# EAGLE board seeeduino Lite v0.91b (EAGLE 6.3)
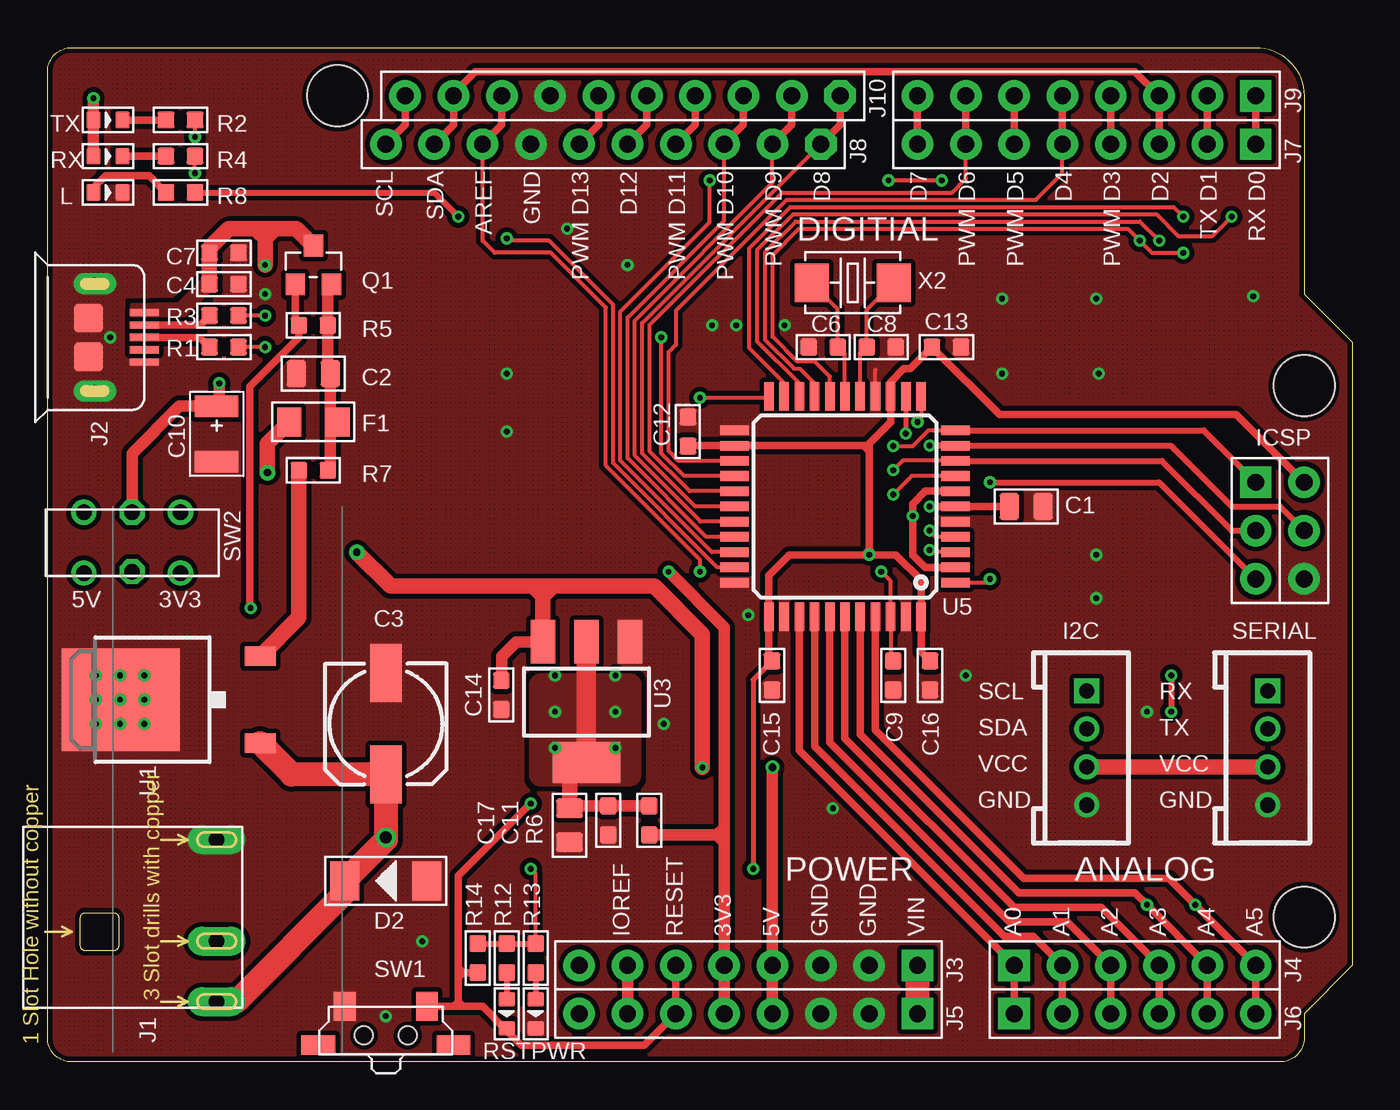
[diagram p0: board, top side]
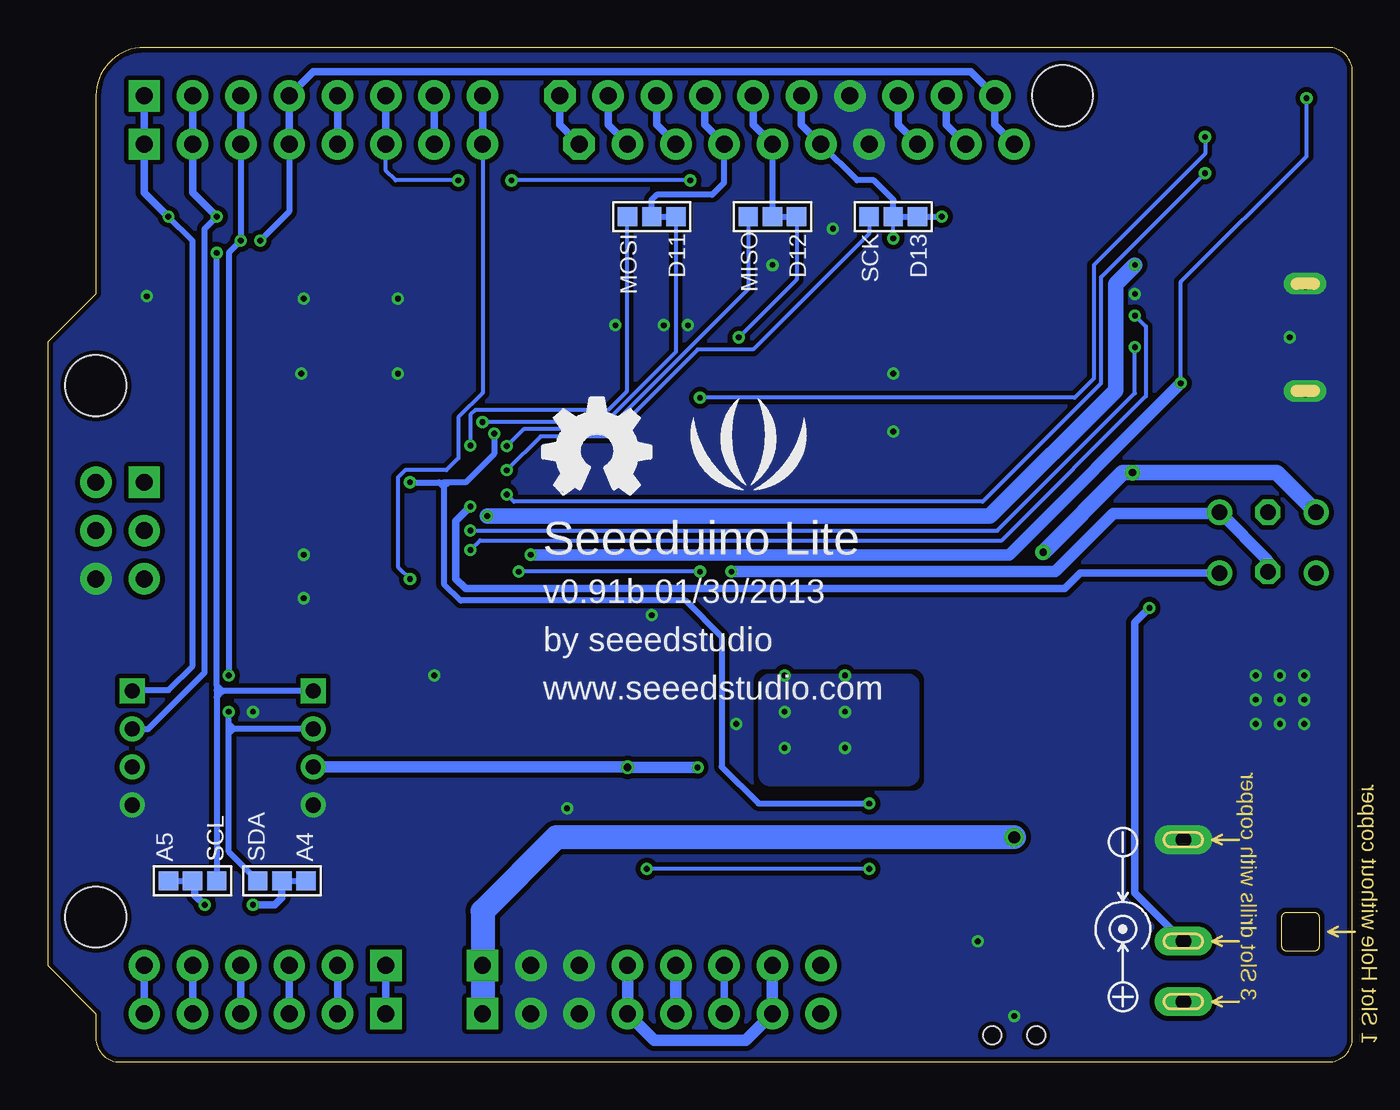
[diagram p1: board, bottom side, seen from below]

Size 68.58 x 53.34 mm. Coordinates in mm from the lower left corner, seen from the top.
Outline: 66.04,2.54 66.04,1.27 arc-90 64.77,0 1.27,0 arc-90 0,1.27 0,52.07 arc-90 1.27,53.34 63.5,53.34 arc-90 66.04,50.8 66.04,40.39 68.58,37.85 68.58,5.08 66.04,2.54
Copper layers (1*16): Top 0.035mm / dielectric 1.5mm / Bottom 0.035mm
Design rules "default *": minimum track width 6mil, minimum drill 12mil, track to track 6mil, track to pad 6mil, pad to pad 6mil, via to via 6mil, smd to smd 0mil, copper to edge 10mil, drill to drill 10mil, minimum pad ring 10mil, minimum via ring 6mil, stop-mask expansion 2mil, vias tented up to drill 100mil, thermal gap 10mil
Net classes: 0 default: width 0.152 mm, drill 0.305 mm, clearance 0.152 mm; 3 none3: width 0.203 mm, drill 0.305 mm, clearance 0.203 mm
Holes 3.2 mm at 15.24,50.8 66.04,35.56 66.04,7.62

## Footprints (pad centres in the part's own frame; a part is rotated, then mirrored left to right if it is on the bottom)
C0805 = smd 1.016 x 1.397: 1 -0.889,0; 2 0.889,0
ELECTRO-SMD-C-6MM = smd 3.048 x 1.651: + 2.667,0; - -2.667,0
C0603 = smd 0.889 x 0.889: 1 -0.762,0; 2 0.762,0
AVX-B = smd 1.143 x 2.286: + -1.46,0; - 1.46,0
D2010 = smd 1.524 x 2.032: + -2.159,0; - 2.159,0
F1206 = smd 1.27 x 1.524: 1 -1.27,0; 2 1.27,0
4P-LEADED-2.0 = drill 0.8 pad 1.27 square: 1 -3,0 | drill 0.8 pad 1.27: 2 -1,0; 3 1,0; 4 3,0
2X3P-2.54 = drill 0.889 pad 1.651 square: 1 -1.27,2.54 | drill 0.889 pad 1.651: 2 -1.27,0; 3 -1.27,-2.54; 4 1.27,-2.54; 5 1.27,0; 6 1.27,2.54
DC-404 = drill 0.813 pad 1.524 long: + 3.175,10.16; - -5.334,10.16; CDN 0,10.16
MICRO-USB-5P = smd 0.38 x 1.52: 1 -1.3,0; 2 -0.65,0; 3 0,0; 4 0.65,0; 5 1.3,0 | smd 1.524 x 1.524: E1 -1.016,-2.921; E2 1.016,-2.921 | drill 0.635 pad 1.143 long: P1 -2.819,-2.591; P2 2.819,-2.591
8P-2.54-65/35MIL = drill 0.889 pad 1.651 square: 1 0,8.89 | drill 0.889 pad 1.651: 2 0,6.35; 3 0,3.81; 4 0,1.27; 5 0,-1.27; 6 0,-3.81; 7 0,-6.35; 8 0,-8.89
6P-2.54-65/35MIL = drill 0.889 pad 1.651 square: 1 0,6.35 | drill 0.889 pad 1.651: 2 0,3.81; 3 0,1.27; 4 0,-1.27; 5 0,-3.81; 6 0,-6.35
10P-2.54 = drill 0.889 pad 1.651 octagon: 1 0,11.43 | drill 0.889 pad 1.651: 2 0,8.89; 3 0,6.35; 4 0,3.81; 5 0,1.27; 6 0,-1.27; 7 0,-3.81; 8 0,-6.35; 9 0,-8.89; 10 0,-11.43
LED-0603 = smd 0.762 x 0.889: + -0.762,0; - 0.762,0
3P-SMD-4.1X1.5 = smd 1.016 x 1.016: 00 -1.27,0; 11 1.27,0; MM 0,0
SOT23 = smd 1.016 x 1.143: 1 -0.95,-1.016; 2 0.95,-1.016; 3 0,1.016
R0603 = smd 0.889 x 0.889: 1 -0.762,0; 2 0.762,0
4P-SMD-7X3.5X3.5H = smd 1.143 x 1.524: 1 -2.159,1.524; 2 2.159,1.524 | smd 1.778 x 1.016: S1 -3.556,-0.508; S2 3.556,-0.508 | hole 0.95: -1.15,0; 1.15,0
6P-2CH-2.5-9.1X3.5X3.2H = drill 0.813 pad 1.27: CH1A -2.54,-1.6; CH1B 2.54,-1.6; CH2A -2.54,1.6; CH2B 2.54,1.6 | drill 0.813 pad 1.27 octagon: COM1 0,-1.6; COM2 0,1.524
TO252 = smd 1.016 x 1.651: 1 -2.286,-4.826; 2 2.286,-4.826 | smd 5.4 x 6.2: 3 0,2.5
SOT-223 = smd 1.27 x 2.286: 1 -2.286,-3.175; 2 0,-3.175; 3 2.286,-3.175 | smd 3.556 x 2.159: TER 0,3.175
TQFP44 = smd 1.5 x 0.5: 1 -5.8,4; 2 -5.8,3.2; 3 -5.8,2.4; 4 -5.8,1.6; 5 -5.8,0.8; 6 -5.8,0; 7 -5.8,-0.8; 8 -5.8,-1.6; 9 -5.8,-2.4; 10 -5.8,-3.2; 11 -5.8,-4; 23 5.8,-4; 24 5.8,-3.2; 25 5.8,-2.4; 26 5.8,-1.6; 27 5.8,-0.8; 28 5.8,0; 29 5.8,0.8; 30 5.8,1.6; 31 5.8,2.4; 32 5.8,3.2; 33 5.8,4 | smd 0.5 x 1.5: 12 -4,-5.8; 13 -3.2,-5.8; 14 -2.4,-5.8; 15 -1.6,-5.8; 16 -0.8,-5.8; 17 0,-5.8; 18 0.8,-5.8; 19 1.6,-5.8; 20 2.4,-5.8; 21 3.2,-5.8; 22 4,-5.8; 34 4,5.8; 35 3.2,5.8; 36 2.4,5.8; 37 1.6,5.8; 38 0.8,5.8; 39 0,5.8; 40 -0.8,5.8; 41 -1.6,5.8; 42 -2.4,5.8; 43 -3.2,5.8; 44 -4,5.8
2P-SMD-5X3.2 = smd 1.778 x 2.032: 1 -2.159,0; 2 2.159,0

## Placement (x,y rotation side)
C1  1uF  [C0805]  51.44,29.21 180 top
C2  10uF  [C0805]  13.97,36.2 180 top
C3  25v_47uF  [ELECTRO-SMD-C-6MM]  17.78,17.78 270 top
C4  100nF  [C0603]  9.27,40.89 0 top
C6  8.2pF  [C0603]  40.77,37.59 0 top
C7  10nF  [C0603]  9.27,42.55 0 top
C8  8.2pF  [C0603]  43.81,37.59 180 top
C9  100nF  [C0603]  44.45,20.32 90 top
C10  47uF 10V  [AVX-B]  8.89,33.02 270 top
C11  100nF  [C0603]  29.46,12.7 90 top
C12  100nF  [C0603]  33.66,33.15 270 top
C13  100nF  [C0603]  47.24,37.59 180 top
C14  100nF  [C0603]  23.85,19.3 90 top
C15  100nF  [C0603]  38.07,20.32 90 top
C16  100nF  [C0603]  46.38,20.32 90 top
C17  10uF  [C0805]  27.43,12.45 90 top
D2  M7  [D2010]  17.78,9.53 180 top
F1  PPTC-500mA  [F1206]  13.97,33.66 180 top
I2C  4P-LEADED-2.0  [4P-LEADED-2.0]  54.61,16.51 270 top
ICSP  2.54-2x3p male  [2X3P-2.54]  64.77,27.94 0 top
J1  DC-044-AH  [DC-404]  -1.27,6.35 270 top
J2  USB-MICRO-5P  [MICRO-USB-5P]  5.08,38.1 270 top
J3  DNP  [8P-2.54-65/35MIL]  36.83,5.08 270 top
J4  DNP  [6P-2.54-65/35MIL]  57.15,5.08 90 top
J5  2.54-6p female  [8P-2.54-65/35MIL]  36.83,2.54 270 top
J6  2.54-6p female  [6P-2.54-65/35MIL]  57.15,2.54 90 top
J7  DNP  [8P-2.54-65/35MIL]  54.61,48.26 270 top
J8  DNP  [10P-2.54]  29.21,48.26 270 top
J9  2.54-8p female  [8P-2.54-65/35MIL]  54.61,50.8 270 top
J10  2.54-8p female  [10P-2.54]  30.23,50.8 270 top
L  GREEN  [LED-0603]  3.17,45.72 0 top
MISO  DNP  [3P-SMD-4.1X1.5]  30.48,44.45 0 bottom
MOSI  DNP  [3P-SMD-4.1X1.5]  36.83,44.45 0 bottom
PWR  GREEN  [LED-0603]  25.65,2.54 270 top
Q1  Si2305Ds  [SOT23]  13.97,41.91 0 top
R1  22R  [R0603]  9.27,37.59 0 top
R2  1k  [R0603]  6.99,49.53 180 top
R3  22R  [R0603]  9.27,39.24 0 top
R4  1k  [R0603]  6.99,47.62 180 top
R5  100k  [R0603]  13.97,38.73 0 top
R6  0R  [R0603]  31.62,12.7 270 top
R7  0R  [R0603]  13.97,31.11 0 top
R8  1k  [R0603]  6.99,45.72 0 top
R12  1k  [R0603]  24.13,5.46 270 top
R13  1k  [R0603]  25.65,5.46 270 top
R14  10k  [R0603]  22.61,5.46 270 top
RST  RED  [LED-0603]  24.13,2.54 270 top
RX  GREEN  [LED-0603]  3.17,47.62 0 top
SCK  DNP  [3P-SMD-4.1X1.5]  24.13,44.45 0 bottom
SCL  DNP  [3P-SMD-4.1X1.5]  60.96,9.53 0 bottom
SDA  DNP  [3P-SMD-4.1X1.5]  56.26,9.53 180 bottom
SERIAL  4P-LEADED-2.0  [4P-LEADED-2.0]  64.14,16.51 270 top
SW1  BUTTON-4P-REINFORCE'TS-118E'  [4P-SMD-7X3.5X3.5H]  17.78,1.4 0 top
SW2  SWITCH-2CH-6P-2.54  [6P-2CH-2.5-9.1X3.5X3.2H]  4.45,27.3 180 top
TX  GREEN  [LED-0603]  3.17,49.53 0 top
U1  78M05-TO252  [TO252]  6.35,19.05 90 top
U3  LD1117S  [SOT-223]  28.32,18.92 180 top
U5  ATMEGA32U4-AU  [TQFP44]  41.91,29.21 180 top
U$1  [OSHW_FILLX200_NOTEXT]  42.55,29.84 0 bottom
U$2  [LOGO_SILK]  31.75,31.75 0 bottom
X2  16MHz  [2P-SMD-5X3.2]  42.32,40.97 180 top

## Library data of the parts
C1-C4 C6-C17 D2 F1 L PWR Q1 R1-R8 R12-R14 RST RX SW1 SW2 TX X2 = Discrete
I2C ICSP J2-J10 SERIAL = Connector
J1 = For_Test_Albert
MISO MOSI SCK SCL SDA = Discrete; PARTNO: DNP
U1 U3 U5 = IC
U$1 U$2 = Logo

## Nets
3V3: J3.5 J5.5 R6.2 SW2.CH1A SW2.COM2
5V [none3]: C14.2 F1.2 I2C.3 J3.4 J3.7 J5.4 J5.7 SERIAL.3 SW2.CH1B U3.3
AREF: C9.2 J8.8 J10.8 U5.42
D14/PB3/MISO: ICSP.1 MISO.00 U5.11
D15/PB1/SCK: ICSP.2 SCK.00 U5.9
D16/PB2/MOSI: ICSP.5 MOSI.00 U5.10
D17/PB0/RXLED: R4.1 U5.8
D+: R1.2 U5.4
D-: R3.2 U5.3
GATE: J1.CDN Q1.1 R5.1
GND [none1]: C1.1 C2.2 C3.- C4.2 C6.1 C7.2 C8.1 C9.1 C10.- C11.1 C12.1 C13.1 C14.1 C15.1 C16.1 C17.1 D2.+ I2C.4 ICSP.4 J1.- J2.5 J2.E1 J2.E2 J2.P1 J2.P2 J3.2 J3.3 J5.2 J5.3 J8.7 J10.7 L.- PWR.- SERIAL.4 SW1.1 U1.3 U3.1 U5.5 U5.15 U5.23 U5.33 U5.35 U5.43
N$1: C6.2 U5.17 X2.2
N$2: C8.2 U5.16 X2.1
N$3: C11.2 C17.2 R6.1 U3.2 U3.TER
N$4: L.+ R8.1
N$5: R2.2 TX.-
N$6: J2.2 R3.1
N$7: R4.2 RX.-
N$8: J2.3 R1.1
N$9: C2.1 F1.1 Q1.2 R5.2 R7.2
N$10: PWR.+ R13.2
N$11: R7.1 U1.2
N$17: R12.2 RST.+
PB4/A8/D8: J8.1 J10.1 U5.28
PB5/A9/D9: J8.2 J10.2 U5.29
PB6/A10/D10: J8.3 J10.3 U5.30
PB7/D11: J8.4 J10.4 MOSI.11 MOSI.MM U5.12
PC7/D13: J8.6 J10.6 R8.2 SCK.11 SCK.MM U5.32
PD0/SCL/D3: I2C.1 J7.4 J8.10 J9.4 J10.10 SCL.11 U5.18
PD1/SDA/D2: I2C.2 J7.3 J8.9 J9.3 J10.9 SDA.11 U5.19
PD2/RXI/D0: J7.1 J9.1 SERIAL.1 U5.20
PD3/TXO/D1: J7.2 J9.2 SERIAL.2 U5.21
PD4/A6/D4: J7.5 J9.5 U5.25
PD5/TXLED: R2.1 U5.22
PD6/A11/D12: J8.5 J10.5 MISO.11 MISO.MM U5.26
PD6/D5: J7.6 J9.6 U5.31
PD7/A7/D6: J7.7 J9.7 U5.27
PE6/D7: J7.8 J9.8 U5.1
PF0/A5: J4.6 J6.6 SCL.00 SCL.MM U5.41
PF1/A4: J4.5 J6.5 SDA.00 SDA.MM U5.40
PF4/A3: J4.4 J6.4 U5.39
PF5/A2: J4.3 J6.3 U5.38
PF6/A1: J4.2 J6.2 U5.37
PF7/A0: J4.1 J6.1 U5.36
PWR_IN: C3.+ D2.- J1.+ J3.1 J5.1 U1.1
RESET: ICSP.3 J3.6 J5.6 R14.2 RST.- SW1.2 U5.13
U5V: C4.1 C7.1 J2.1 Q1.3 U5.2 U5.7
UCAP: C1.2 SW2.CH2A U5.6
VCC: C10.+ C12.2 C13.2 C15.2 C16.2 ICSP.6 R12.1 R13.1 R14.1 RX.+ SW2.COM1 TX.+ U5.14 U5.24 U5.34 U5.44

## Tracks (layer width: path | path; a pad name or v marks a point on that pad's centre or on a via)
3V3  (via drill 0.3 pad 0.64)
  Top 0.61: J5.5 J3.5 35.56,11.56 | v32.64,25.78 35.56,22.86 35.56,12.32 | 35.56,11.81 35.56,12.32 | R6.2 35.18,11.94 | 35.18,11.94 35.43,11.94 35.56,11.81 | 35.18,11.94 35.56,12.32 | 35.18,11.94 35.56,11.56 | 35.56,11.56 35.56,11.81
  Bottom 0.61: SW2.COM2 4.45,26.36 SW2.CH1A arc90 7.06,28.83 12.57,28.83 15.62,25.78 v32.64,25.78 | J5.5 J3.5
5V  (via drill 0.3 pad 0.64, 0.38 pad 0.81, 0.41)
  Top 0.61: J5.4 J3.4 v38.1,15.49 | U3.3 24.64,22.1 23.88,21.34 23.88,20.09 C14.2 | J3.7 J5.7
  Top 0.813: SERIAL.3 I2C.3 | F1.2 11.56,32.51 v11.56,30.99 | v16.26,26.8 18.03,25.02 25.53,25.02 | 25.53,25.02 26.16,25.02 | 26.16,25.02 26.04,24.89 26.04,24.51 | 26.04,24.51 26.04,24.38 | 26.04,24.38 U3.3 | 26.04,24.38 arc45 25.95,24.6 25.53,25.02 | 26.16,25.02 31.88,25.02 34.42,22.48 v34.42,15.49 | 26.04,24.51 26.42,24.89
  Bottom 0.61: I2C.3 38.12,15.51 v38.1,15.49 v34.42,15.49 | J5.7 31.88,1.14 36.7,1.14 J5.4 J3.4 | J3.7 30.48,2.67
  Bottom 0.813: SW2.CH1B 3.99,30.99 v11.56,30.99 12.06,30.99 v16.26,26.8
AREF  (via drill 0.3 pad 0.64)
  Top 0.203: 44.31,21.22 U5.42 44.31,25.29 v43.81,25.78 | J8.8 22.86,43.18 23.5,42.55 26.46,42.55 29.34,39.67 29.34,31.37 34.29,26.42 v34.29,25.78
  Top 0.305: 44.31,21.22 C9.2
  Top 0.406: J10.8 23.88,49.28 J8.8
  Bottom 0.203: v34.29,25.78 v43.81,25.78
  Bottom 0.406: J10.8 23.88,49.28 J8.8
D14/PB3/MISO  (via drill 0.3 pad 0.64)
  Top 0.203: 47.65,33.27 U5.11 46.29,33.21 45.47,32.38 v44.45,32.38
  Top 0.305: U5.11 60.77,33.21 ICSP.1
  Bottom 0.203: MISO.00 31.75,40.64 39.12,33.27 43.56,33.27 v44.45,32.38
D15/PB1/SCK  (via drill 0.3 pad 0.64)
  Top 0.203: 47.57,31.75 47.7,31.62 | 47.7,31.62 U5.9 | 47.7,31.62 44.96,31.62 v44.45,31.11
  Top 0.305: U5.9 58.56,31.61 62.23,27.94 ICSP.2
  Bottom 0.203: 25.4,44.07 SCK.00 25.4,43.56 31.5,37.47 34.42,37.47 38.99,32.89 42.67,32.89 v44.45,31.11
D16/PB2/MOSI  (via drill 0.3 pad 0.64)
  Top 0.305: U5.10 v46.35,32.41 59.03,32.41 62.23,29.21 64.77,29.21 ICSP.5
  Bottom 0.203: MOSI.00 arc-45 38.14,44.43 38.14,35.26 39.12,34.29 46.1,34.29 46.35,34.04 v46.35,32.41
D17/PB0/RXLED  (via drill 0.3 pad 0.64)
  Top 0.203: U5.8 45.41,30.81 v44.45,29.84 | v7.75,46.74 R4.1
  Bottom 0.203: v44.45,29.84 44.07,29.46 19.43,29.46 13.21,35.69 13.21,41.27 v7.75,46.74
D+  (via drill 0.3 pad 0.64)
  Top 0.203: U5.4 46.69,27.61 v46.35,27.94 | v11.43,37.59 R1.2
  Bottom 0.203: v46.35,27.94 18.66,27.94 11.43,35.17 v11.43,37.59
D-  (via drill 0.3 pad 0.64)
  Top 0.203: U5.3 46.47,26.81 v46.35,26.92 | v11.43,39.24 R3.2
  Bottom 0.203: v46.35,26.92 45.85,27.43 18.43,27.43 10.86,35 10.86,38.67 v11.43,39.24
GATE  (via drill 0.3 pad 0.64)
  Top 0.406: Q1.1 13.02,38.92 R5.1 | R5.1 13.08,38.73 | R5.1 13.21,38.1 10.63,35.52 10.63,23.91 v10.67,23.88
  Bottom 0.406: J1.CDN 11.43,8.89 11.43,23.11 v10.67,23.88
GND  (via drill 0.3 pad 0.64)
  Top 0.203: U5.15 43.51,36.4
  other vias: 50.16,36.2 55.24,36.2 50.16,40.13 41.27,13.34 36.83,23.5 11.43,40.39 30.48,41.91 57.78,18.41 55.12,40.13 63.37,40.26 24.13,36.2 24.13,33.15 3.3,38.1 19.68,6.35 17.78,2.41 48.26,20.32 55.12,26.67 55.12,24.38 32.38,17.78 34.92,38.73 2.54,20.32 5.08,20.32 5.08,17.78 2.54,17.78 27.3,43.81 38.73,38.73 36.2,38.73 5.08,19.05 2.54,19.05 3.81,20.32 3.81,19.05 3.81,17.78
  pour Bottom (isolate 0.254, rank 2, no thermals): 0,0 66.04,0 66.04,2.54 68.58,5.08 68.58,37.85 66.04,40.39 66.04,51.82 64.52,53.34 0,53.34
  pour Top (isolate 0.254, rank 2, no thermals, hatched): 0,0 66.04,0 66.04,2.54 68.58,5.08 68.58,37.85 66.04,40.39 66.04,51.82 64.52,53.34 0,53.34
N$1
  Top 0.203: X2.2 41.53,39.6 C6.2 41.91,37.21 U5.17
N$2
  Top 0.203: U5.16 42.71,37.25 C8.2 43.05,39.55 X2.1
N$3  (via drill 0.3 pad 0.64)
  Top 0.305: 27.43,15.62 28.19,15.62 U3.TER
  Top 0.61: C17.2 27.56,13.46 C11.2 R6.1
  Top 0.813: C17.2 27.43,15.62
  Top 1.016: U3.TER U3.2
  other vias: 26.67,20.32 26.67,16.51 29.84,16.51 29.84,18.41 26.67,18.41 29.84,20.32
  pour Bottom (isolate 0.254, no thermals): 22.86,19.81 22.86,15.11 arc90 23.37,14.61 30.61,14.61 arc90 31.11,15.11 31.11,19.81 arc90 30.61,20.32 23.37,20.32 arc90
  pour Top (isolate 0.254, no thermals): 25.4,19.81 25.4,15.11 arc90 25.91,14.61 30.61,14.61 arc90 31.11,15.11 31.11,19.81 arc90 30.61,20.32 25.91,20.32 arc90
N$4
  Top 0.406: L.+ 2.41,45.97 3.05,46.61 5.33,46.61 R8.1
N$5
  Top 0.406: TX.- R2.2
N$6
  Top 0.406: J2.2 8.02,38.75 R3.1
N$7
  Top 0.406: R4.2 RX.-
N$8
  Top 0.406: J2.3 8,38.1 R1.1
N$9
  Top 0.406: 14.92,38.92 R5.2 | 14.86,34.04 F1.1
  Top 0.61: Q1.2 14.73,40.89 R5.2 14.73,36.32 C2.1 14.86,34.04 14.86,31.24 R7.2
N$10
  Top 0.305: R13.2 PWR.+
N$11
  Top 0.813: R7.1 13.21,23.37 U1.2
N$17
  Top 0.305: R12.2 RST.+
PB4/A8/D8
  Top 0.203: U5.28 34.04,29.21 31.24,32 31.24,38.86 J8.1 40.51,48.26
  Top 0.406: J10.1 41.66,49.28 J8.1
  Bottom 0.406: J10.1 41.66,49.28 J8.1
PB5/A9/D9
  Top 0.203: U5.29 34.33,28.41 30.86,31.88 30.86,38.99 38.1,46.23 J8.2
  Top 0.406: J10.2 39.12,49.28 J8.2
  Bottom 0.406: J10.2 39.12,49.28 J8.2
PB6/A10/D10
  Top 0.203: U5.30 34.62,27.61 30.48,31.75 30.48,39.15 35.56,44.23 J8.3
  Top 0.406: J10.3 36.58,49.28 J8.3
  Bottom 0.406: J10.3 36.58,49.28 J8.3
PB7/D11  (via drill 0.3 pad 0.64)
  Top 0.203: U5.12 45.91,33.84 v45.72,33.66
  Top 0.406: J10.4 34.04,49.28 J8.4
  Bottom 0.203: MOSI.11 35.56,37.34 39.24,33.66 v45.72,33.66
  Bottom 0.305: MOSI.11 MOSI.MM 36.83,45.34 36.58,45.59 33.66,45.59 33.02,46.23 J8.4
  Bottom 0.406: J10.4 34.04,49.28 J8.4
PC7/D13  (via drill 0.3 pad 0.64)
  Top 0.203: U5.32 35.2,26.01 29.72,31.5 29.72,39.83 26.36,43.18 24.26,43.18 v24.13,43.31
  Top 0.305: R8.2 20.32,45.72 v21.59,44.45
  Top 0.406: J10.6 28.96,49.28 J8.6
  Bottom 0.203: v24.13,43.31 SCK.MM
  Bottom 0.305: J8.6 26.04,46.35 25.15,46.35 24.13,45.33 SCK.MM SCK.11 v21.59,44.45
  Bottom 0.406: J10.6 28.96,49.28 J8.6
PD0/SCL/D3  (via drill 0.3 pad 0.64)
  Top 0.203: U5.18 41.11,36.05 40.33,36.83 39.41,36.83 38.1,38.13 38.1,42.43 39.49,43.81 56.77,43.81 v57.4,43.18 58.04,42.55 v59.69,42.55
  Top 0.406: J9.4 J7.4 | J10.10 18.8,49.28 J8.10
  Bottom 0.305: 59.69,19.81 59.69,19.56 | 59.69,19.56 59.69,19.18 | 59.69,19.18 SCL.11 | I2C.1 59.39,19.51 | 59.39,19.51 59.64,19.51 59.69,19.56 | 59.39,19.51 59.39,19.52 59.69,19.81 | 59.39,19.51 59.39,19.47 59.69,19.18 | 59.69,19.81 v59.69,42.55 | J7.4 55.88,44.7 v57.4,43.18
  Bottom 0.406: J8.10 18.8,49.28 J10.10 20.07,52.07 54.61,52.07 J9.4 J7.4
PD1/SDA/D2  (via drill 0.3 pad 0.64)
  Top 0.203: U5.19 40.26,35.06 40.26,35.73 39.54,36.45 39.24,36.45 37.7,37.99 37.7,42.58 39.32,44.2 57.4,44.2 v58.42,43.18
  Top 0.305: v59.05,20.32 v59.05,18.41
  Top 0.406: J7.3 J9.3 57.15,52.07 22.48,52.07 21.34,50.93 J10.9 21.34,49.28 J8.9
  Bottom 0.305: SDA.11 57.66,9.53 57.66,9.65 59.05,11.05 59.05,17.27 | v59.05,20.32 59.05,42.55 v58.42,43.18 J7.3 | 59.05,17.27 59.05,17.53 | 59.05,17.53 59.05,17.78 | 59.05,17.78 v59.05,18.41 | I2C.2 58.78,17.51 | 58.82,17.51 59.04,17.51 59.05,17.53 | 58.78,17.51 59.05,17.78 | 58.78,17.51 58.82,17.51 | 58.82,17.51 59.05,17.27
  Bottom 0.406: J10.9 21.34,49.28 J8.9 | J9.3 J7.3
PD2/RXI/D0  (via drill 0.3)
  Top 0.203: U5.20 39.5,35.02 39.5,35.69 37.28,37.9 37.28,42.68 39.18,44.58 58.29,44.58 59.44,43.43 61.21,43.43 v62.23,44.45
  Top 0.406: J9.1 J7.1
  Bottom 0.305: SERIAL.1 64.09,19.56 62.23,19.56 60.96,20.83 60.96,43.18 v62.23,44.45
  Bottom 0.406: J9.1 J7.1 63.5,45.72 v62.23,44.45
PD3/TXO/D1  (via drill 0.3 pad 0.64)
  Top 0.203: U5.21 38.86,35.16 38.86,35.56 36.89,37.54 36.89,42.8 39.04,44.96 59.18,44.96 v59.69,44.45
  Top 0.406: J9.2 J7.2
  Bottom 0.305: SERIAL.2 63.29,17.51 60.33,20.48 60.33,43.81 v59.69,44.45
  Bottom 0.406: J9.2 J7.2 60.96,45.72 v59.69,44.45
PD4/A6/D4
  Top 0.203: U5.25 33.16,31.61 32.64,32.13 32.64,37.34 33.02,37.72 33.02,39.5 38.86,45.34 51.94,45.34 53.34,46.74 J7.5
  Top 0.406: J9.5 J7.5
  Bottom 0.406: J7.5 J9.5
PD5/TXLED  (via drill 0.3 pad 0.64)
  Top 0.203: 37.97,35.56 37.97,35.07 U5.22 37.83,34.92 v34.29,34.92 | R2.1 v7.75,48.64
  Bottom 0.203: v7.75,48.64 7.75,47.75 13.59,41.91 13.59,35.94 14.61,34.92 v34.29,34.92
PD6/A11/D12  (via drill 0.3 pad 0.64)
  Top 0.203: U5.26 33.45,30.81 32.26,32 v32.26,38.1
  Top 0.406: J10.5 31.5,49.28 J8.5
  Bottom 0.203: MISO.11 29.21,41.15 v32.26,38.1
  Bottom 0.305: MISO.11 MISO.MM J8.5
  Bottom 0.406: J10.5 31.5,49.28 J8.5
PD6/D5  (via drill 0.3 pad 0.64)
  Top 0.203: U5.31 34.91,26.81 30.1,31.62 30.1,39.46 34.8,44.16 v34.8,46.35 | v44.2,46.35 v46.99,46.35
  Top 0.406: J9.6 J7.6
  Bottom 0.203: v34.8,46.35 v44.2,46.35 | v46.99,46.35 50.29,46.35 50.8,46.86 J7.6
  Bottom 0.406: J9.6 J7.6
PD7/A7/D6
  Top 0.203: U5.27 33.74,30.01 31.62,32.13 31.62,38.73 38.61,45.72 47.54,45.72 48.26,46.44 J7.7
  Top 0.406: J9.7 J7.7
  Bottom 0.406: J9.7 J7.7
PE6/D7  (via drill 0.3 pad 0.64)
  Top 0.203: U5.1 49.34,25.21 v49.53,25.4
  Top 0.406: J9.8 J7.8
  Bottom 0.203: J7.8 45.72,35.18 46.99,33.91 46.99,31.75 47.62,31.11 49.78,31.11 50.16,30.73 50.16,26.04 v49.53,25.4
  Bottom 0.406: J9.8 J7.8
PF0/A5  (via drill 0.3 pad 0.64)
  Top 0.406: J6.6 J4.6 v60.33,8.26 58.93,9.65 51.31,9.65 43.51,17.45 U5.41
  Bottom 0.305: SCL.00 SCL.MM
  Bottom 0.406: SCL.MM 60.83,9.4 60.83,8.76 v60.33,8.26 | J6.6 J4.6
PF1/A4  (via drill 0.3 pad 0.64)
  Top 0.406: J6.5 J4.5 v57.78,8.26 57.15,8.89 51.05,8.89 42.71,17.23 U5.40
  Bottom 0.305: SDA.MM SDA.00
  Bottom 0.406: SDA.MM 56.26,8.64 56.64,8.26 v57.78,8.26 | J6.5 J4.5
PF4/A3
  Top 0.406: J6.4 J4.4 55.37,8.13 50.8,8.13 41.91,17.02 U5.39
  Bottom 0.406: J6.4 J4.4
PF5/A2
  Top 0.406: J6.3 J4.3 53.59,7.37 50.55,7.37 41.11,16.8 U5.38
  Bottom 0.406: J6.3 J4.3
PF6/A1
  Top 0.406: J6.2 J4.2 51.82,6.6 50.29,6.6 40.31,16.59 U5.37
  Bottom 0.406: J6.2 J4.2
PF7/A0
  Top 0.406: J6.1 J4.1 39.51,16.37 U5.36
  Bottom 0.406: J6.1 J4.1
PWR_IN  (via drill 0.64 pad 1.02)
  Top 1.27: J1.+ 9.91,3.17 15.75,9.02 15.75,9.14 15.49,9.4 D2.- 17.78,11.68 v17.78,11.81 C3.+ 12.83,15.11 U1.1 | J3.1 J5.1
  Bottom 1.27: v17.78,11.81 41.83,11.81 45.72,7.92 J3.1 J5.1
RESET  (via drill 0.3 pad 0.64)
  Top 0.254: U5.13 v45.11,33.05
  Top 0.305: v49.53,30.48 58.42,30.48 ICSP.3
  Top 0.406: 45.09,34.98 U5.13 | J3.6 J5.6 31.37,0.89 24.89,0.89 24.13,1.65 | RST.- 24.13,1.65 | SW1.2 21.34,2.92 | 21.34,2.92 21.59,2.92 | 21.59,4.95 21.59,9.78 v25.4,13.59 | 21.59,4.95 21.59,4.7 | 21.59,4.7 21.59,4.45 | 21.59,4.45 21.59,3.17 | 21.59,3.17 21.59,2.92 | R14.2 21.84,4.7 | 21.84,4.7 21.59,4.7 | 21.59,2.92 21.84,2.92 | 21.84,2.92 22.86,2.92 24.13,1.65 | 21.34,2.92 21.59,3.17 | 21.59,3.17 21.84,2.92 | 21.84,4.7 21.59,4.95 | 21.84,4.7 21.59,4.45
  Bottom 0.305: v25.4,13.59 31.21,13.59 33.15,15.53 33.15,22.35 35.05,24.26 46.86,24.26 47.75,25.15 47.75,30.23 | 47.75,30.48 47.75,30.23 | v49.53,30.48 48.01,30.48 | 48.01,30.48 47.75,30.48 | v45.11,33.05 45.11,31.98 46.61,30.48 47.5,30.48 | 47.5,30.48 47.75,30.48 | 47.75,30.23 47.5,30.48 | 47.75,30.23 48.01,30.48
  Bottom 0.406: J3.6 33.02,2.67
U5V  (via drill 0.3 pad 0.64)
  Top 0.406: U5.7 46.14,30.01 45.47,29.34 v45.47,28.7 45.47,26.67 46.13,26.01 U5.2 | C7.1 8.51,42.8
  Top 0.813: Q1.3 13.08,43.81 11.43,43.81 | C4.1 C7.1 | 11.43,43.81 11.43,43.31 | 11.43,43.31 v11.43,41.91 | 11.43,43.81 9.53,43.81 8.51,42.8 | 11.43,43.31 11.05,43.69 | 11.43,43.31 11.81,43.69
  Bottom 0.813: v11.43,41.91 12.45,40.89 12.45,35.31 19.05,28.7 v45.47,28.7
  pour Top (no thermals): 4.39,39.24 7.24,39.24 8.64,40.64 8.64,41.15 8.13,41.15 6.86,39.88 4.39,39.83
UCAP  (via drill 0.3 pad 0.64)
  Top 0.406: C1.2 U5.6 v46.35,29.21
  Bottom 0.406: SW2.CH2A 14.3,25.7 15.11,24.89 46.61,24.89 47.12,25.4 47.12,28.45 v46.35,29.21
VCC  (via drill 0.3 pad 0.64)
  Top 0.203: R13.1 25.65,9.91 v25.4,10.16
  Top 0.254: C15.2 37.08,20.09 v37.08,10.16 | 24,6.35 R12.1
  Top 0.305: R13.1 R12.1 R14.1
  Top 0.406: C16.2 45.91,21.55 U5.44 45.91,25.34 44.58,26.67 43.43,26.67 | C15.2 37.91,21.25 U5.34 37.91,25.59 38.99,26.67 42.93,26.67 | C12.2 33.68,32.41 U5.24 43.08,32.41 43.18,32.51 | 44.32,35 U5.14 | U5.14 44.31,35.75 45.01,36.45 45.34,36.45 C13.2 50.04,34.04 62.48,34.04 ICSP.6 | 43.43,26.67 v43.18,26.67 | v43.18,26.67 43.18,26.92 | 43.18,26.92 43.18,32.13 | 43.18,32.13 43.18,32.51 | U5.14 44.31,33.64 43.18,32.51 | 43.18,32.13 42.93,32.38 | 42.93,26.67 v43.18,26.67 | 42.93,26.67 43.18,26.92 | 43.43,26.67 43.18,26.92
  Top 0.61: R13.1 25.78,6.22 | RX.+ TX.+ v2.41,50.67 | SW2.COM1 4.45,32 6.92,34.48 C10.+ 9.02,34.61 v9.02,35.69
  Bottom 0.203: v9.02,35.69 9.02,41.02 RX.+ v2.41,50.67 | v25.4,10.16 v37.08,10.16
  Bottom 0.61: v43.18,26.67 18.03,26.67 v9.02,35.69

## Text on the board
tPlace: SCL | SDA | AREF | GND | PWM D13 | D12 | PWM D11 | PWM D10 | PWM D9 | D8 | D7 | PWM D6 | PWM D5 | D4 | PWM D3 | D2 | TX D1 | RX D0 | DIGITIAL | 5V | 3V3 | SCL | RX | SDA | TX | VCC | VCC | GND | GND | POWER | ANALOG | IOREF | RESET | 3V3 | 5V | GND | GND | VIN | A0 | A1 | A2 | A3 | A4 | A5
bPlace: D13 | SCK | D12 | D11 | MOSI | Seeeduino Lite | v0.91b 01/30/2013 | by seeedstudio | www.seeedstudio.com | A4 | SDA | SCL | A5
tValues: Valid combinations: | 3.3V Reg / 8MHz | 5V Reg / 16MHz | Mark back accordingly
